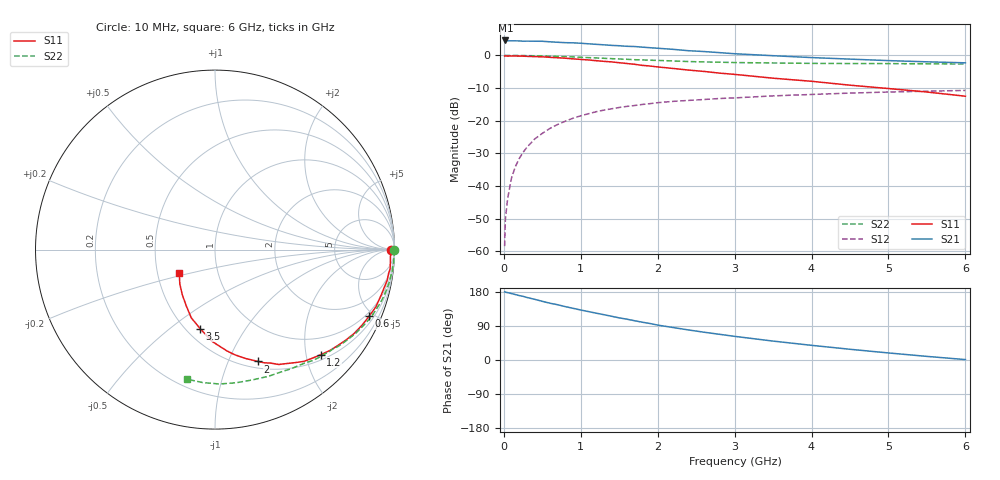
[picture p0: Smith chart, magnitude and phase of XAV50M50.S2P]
! SIEMENS Discrete & RF Semiconductors
! BFY180
! Si NPN RF Bipolar Junction Transistor in MICRO-X
! VCE = 0.5 V  IC = 0.5 mA
! Common Emitter S-Parameters:  May  1997
# GHz  S  MA  R  50
!  f  S11  S21  S12  S22
! GHz  MAG  ANG  MAG  ANG  MAG  ANG  MAG  ANG
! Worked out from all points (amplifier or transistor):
!   36 points, 10 MHz to 6 GHz, reference 50 ohm
!   highest |S21| = 4.6 dB at 20 MHz (marker M1)
!   |S21| within 3 dB of that: start of sweep to 2.334 GHz
!   unconditionally stable (mu >= 1): 3.471 GHz to end of sweep
!   at 250 MHz: K = 0.07, MSG = 17.0 dB, |S12| = -29.7 dB
!   at 1.4 GHz: K = 0.52, MSG = 9.7 dB, |S12| = -16.3 dB
!   at 6 GHz: K = 1.15, MAG = 1.9 dB, |S12| = -10.7 dB
!   S11 on the Smith chart (normalised r, x): 10 MHz: 95, -16; 600 MHz: 0.79, -4.70; 1.2 GHz: 0.61, -2.29; 2 GHz: 0.57, -1.29; 3.5 GHz: 0.58, -0.64; 6 GHz: 0.65, -0.18
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0.01  0.9797 -0.2  1.662 179.9  0.0012 88.1  0.9964 -0.2
0.02  0.9797 -0.9  1.695 179.0  0.0031 95.9  0.9999 -0.5
0.05  0.9783 -2.0  1.674 177.8  0.0065 86.3  0.9992 -1.3
0.1  0.9795 -4.0  1.673 175.2  0.0133 87.5  0.9974 -2.8
0.15  0.9815 -6.3  1.672 172.7  0.0198 86.6  0.9974 -4.0
0.2  0.976 -7.9  1.667 170.0  0.0263 84.5  0.9963 -5.3
0.3  0.9681 -12.0  1.656 165.0  0.0392 80.3  0.9913 -8.1
0.4  0.959 -15.7  1.65 160.2  0.0524 77.7  0.9881 -10.6
0.6  0.9353 -23.4  1.616 149.8  0.0764 71.2  0.9743 -15.9
0.9  0.8863 -34.7  1.559 136.4  0.1093 62.4  0.9477 -23.2
1.1  0.852 -41.3  1.506 127.8  0.128 57.2  0.9254 -27.8
1.2  0.8307 -44.8  1.479 123.6  0.1374 54.4  0.9148 -30.2
1.5  0.7733 -54.5  1.407 111.2  0.1596 47.5  0.8824 -36.2
1.7  0.7319 -61.0  1.369 103.6  0.171 43.5  0.8598 -39.9
2  0.6668 -69.1  1.288 92.1  0.1889 38.3  0.8386 -45.2
2.2  0.6315 -74.1  1.239 85.7  0.1979 34.4  0.8233 -48.7
2.6  0.569 -83.2  1.147 73.4  0.2113 29.0  0.7956 -54.5
2.8  0.5362 -87.7  1.104 67.9  0.2189 26.4  0.7876 -57.5
3.5  0.4481 -100.7  0.99 49.9  0.2401 18.6  0.7661 -67.1
4.5  0.3502 -117.4  0.878 28.3  0.2649 8.1  0.7512 -81.0
5.5  0.2753 -135.3  0.798 9.5  0.2833 -2.0  0.744 -95.3
6  0.2371 -147.4  0.77 1.1  0.291 -7.0  0.7386 -102.4
